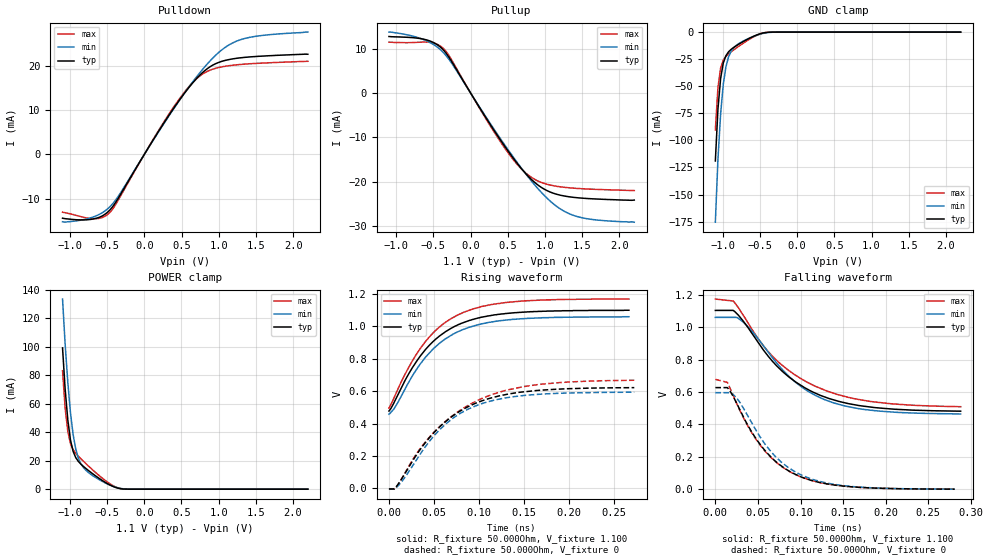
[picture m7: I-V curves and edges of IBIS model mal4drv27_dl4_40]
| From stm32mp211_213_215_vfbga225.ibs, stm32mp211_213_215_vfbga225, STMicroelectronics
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[Model] mal4drv27_dl4_40
Model_type   I/O
Polarity   Non-Inverting
Enable   Active-High
C_comp   1.656pF   1.654pF   1.662pF
C_comp_pullup   832.475fF   825.290fF   839.619fF
C_comp_pulldown 737.556fF   736.745fF   750.731fF
Vinh = 366.000mV
Vinl = 246.000mV
Vmeas = 306.000mV
Vref = 0.00V
Rref = 50Ohms
Cref = 0pF
[Model Spec]
Vinh   366.000mV   354.000mV   385.000mV
Vinl   246.000mV   234.000mV   265.000mV
Vmeas   306.000mV   294.000mV   325.000mV
Vref   0.00V   0.00V   0.00V
D_overshoot_ampl_h 0.3 NA   NA
D_overshoot_ampl_l 0.3 NA   NA
D_overshoot_area_l 100.000m NA   NA
D_overshoot_area_h 100.000m NA   NA
[Receiver Thresholds]
Vth = 306.000mV
Vth_min = 294.000mV
Vth_max = 325.000mV
Vinh_ac = 600.000mV
Vinh_dc = 600.000mV
Vinl_ac = -600.000mV
Vinl_dc = -600.000mV
Tslew_ac = 5.000ns
Threshold_sensitivity = 0.5
Reference_supply Pullup_ref
[Temperature Range]   25.000   125.000   -40.000
[Voltage Range]   1.100V   1.060V   1.170V
[GND Clamp Reference]   0.00V   0.00V   0.00V
[C Comp Corner]
| variable   typ   min   max
C_comp 1.662pF   1.656pF   1.654pF
C_comp_pullup 832.475fF   839.619fF   825.290fF
C_comp_pulldown 736.745fF   750.731fF   737.556fF
[Pulldown Reference]   0.00V   0.00V   0.00V
[POWER Clamp Reference]   1.100V   1.060V   1.170V
[Pullup Reference]   1.100V   1.060V   1.170V
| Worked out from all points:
|   slope of the pulldown table from 0 to 0.165 V, typ, clamps not added: 36.7 ohm
|   slope of the pullup table from 0 to 0.165 V, typ, clamps not added: 36.7 ohm
|   GND clamp passes 1 mA (typ) near -0.47 V on its own axis
|   POWER clamp passes 1 mA (typ) near -0.37 V on its own axis
|   rising waveform, R_fixture 50.000Ohm, V_fixture 1.100: 20-80 % time 53.2ps typ, 53ps min, 53.8ps max; typ from 0.478 V to 1.1 V
|   rising waveform, R_fixture 50.000Ohm, V_fixture 0: 20-80 % time 64.3ps typ, 59.5ps min, 73.7ps max; typ from -0.003 V to 0.622 V
|   falling waveform, R_fixture 50.000Ohm, V_fixture 1.100: 20-80 % time 71.3ps typ, 67.2ps min, 77.8ps max; typ from 1.1 V to 0.481 V
|   falling waveform, R_fixture 50.000Ohm, V_fixture 0: 20-80 % time 54.5ps typ, 54.4ps min, 54.9ps max; typ from 0.627 V to 0.001 V
[GND Clamp]
-1.099V   -119mA     -175.5mA   -90.46mA
-1.064V   -70.81mA   -117.3mA   -51.1mA
-1.028V   -42.76mA   -75.52mA   -33.21mA
-992.7mV  -28.64mA   -48.36mA   -25.94mA
-957.3mV  -21.83mA   -32.18mA   -22.47mA
-921.8mV  -18.22mA   -22.95mA   -20.16mA
-886.4mV  -15.9mA    -17.64mA   -18.21mA
-815.5mV  -12.5mA    -12.17mA   -14.62mA
-567.3mV  -3.324mA   -3.512mA   -3.774mA
-460.9mV  -879.1uA   -1.269mA   -863.6uA
-390mV    -181.5uA   -432.7uA   -123.2uA
2.198V    31.48nA    451.7nA    3.508nA
[Power Clamp]
-1.098V   99.1mA     133.3mA    83.09mA
-1.063V   70.06mA    101.6mA    56.85mA
-1.027V   48.48mA    74.82mA    40.4mA
-991.8mV  34.54mA    53.74mA    31.95mA
-956.4mV  26.58mA    38.45mA    27.74mA
-920.9mV  22.17mA    28.22mA    25.15mA
-885.5mV  19.46mA    21.74mA    23.1mA
-814.5mV  15.82mA    14.94mA    19.43mA
-743.6mV  12.83mA    11.41mA    15.93mA
-460mV    2.904mA    2.84mA     3.733mA
-282.7mV  117.7uA    274uA      108uA
2.199V    -10.68nA   -391.6nA   -2.283nA
[Pulldown]
-1.099V   -14.4mA    -15.2mA    -13.04mA
-673.6mV  -14.53mA   -14.04mA   -14.52mA
-567.3mV  -13.91mA   -13.19mA   -14.26mA
-460.9mV  -12.52mA   -11.78mA   -13.07mA
-319.1mV  -9.014mA   -8.658mA   -9.388mA
141.8mV   3.877mA    3.782mA    4.016mA
460.9mV   12mA       11.92mA    12.29mA
673.6mV   16.59mA    16.87mA    16.63mA
886.4mV   19.81mA    21.15mA    19.03mA
1.099V    21.26mA    24.3mA     19.92mA
1.312V    21.83mA    25.99mA    20.32mA
2.198V    22.6mA     27.6mA     21.01mA
[Pullup]
-1.098V   12.8mA     13.8mA     11.52mA
-637.3mV  12.21mA    12.14mA    11.54mA
-495.5mV  11.41mA    10.95mA    11.31mA
-389.1mV  10.15mA    9.549mA    10.43mA
-282.7mV  7.886mA    7.442mA    8.268mA
213.6mV   -5.793mA   -5.596mA   -6.04mA
532.7mV   -13.8mA    -13.53mA   -14.18mA
745.5mV   -18.3mA    -18.38mA   -18.15mA
958.2mV   -21.42mA   -22.61mA   -20.25mA
1.206V    -23.1mA    -26.21mA   -21.2mA
1.419V    -23.65mA   -27.86mA   -21.55mA
2.199V    -24.2mA    -29.2mA    -22.05mA
[Ramp]
R_load=50.000Ohm
dV/dt_r   373.440mV/59.500ps  357.809mV/57.500ps  400.680mV/65.500ps
dV/dt_f   373.440mV/64.500ps  357.809mV/62.500ps  400.680mV/68.000ps
[Rising waveform]
R_fixture=50.000Ohm
V_fixture=1.100
V_fixture_min=1.060
V_fixture_max=1.170
0s        477.8mV    458.7mV    496.4mV
9ps       568.3mV    521.4mV    602.3mV
20ps      688.3mV    635.9mV    727.2mV
30ps      779.2mV    729.7mV    823.4mV
39ps      846.3mV    798.5mV    895.4mV
60ps      956.3mV    912mV      1.014V
82ps      1.022V     980mV      1.085V
110ps     1.065V     1.024V     1.131V
148ps     1.088V     1.048V     1.157V
267ps     1.1V       1.06V      1.169V
[Rising waveform]
R_fixture=50.000Ohm
V_fixture=0
0s        -2.708mV   -4.143mV   -2.859mV
7ps       3.784mV    177.8uV    -2.859mV
15ps      66.75mV    47.29mV    68.05mV
33ps      227.4mV    198mV      233mV
57ps      383.6mV    365.8mV    385.3mV
76ps      466.6mV    452mV      470.7mV
96ps      525.2mV    509.1mV    536.2mV
128ps     577.9mV    557.5mV    603mV
166ps     605.4mV    581mV      641.9mV
273ps     622.3mV    594.2mV    668.1mV
[Falling waveform]
R_fixture=50.000Ohm
V_fixture=1.100
V_fixture_min=1.060
V_fixture_max=1.170
0s        1.103V     1.06V      1.173V
21ps      1.103V     1.06V      1.161V
32ps      1.042V     1.034V     1.08V
50ps      906.5mV    929.7mV    930.6mV
67ps      789.4mV    811.2mV    820.3mV
93ps      665.8mV    664.7mV    707mV
116ps     595.9mV    582.3mV    638.2mV
137ps     553.8mV    535.4mV    594.9mV
174ps     512.3mV    492.4mV    548.4mV
288ps     481.4mV    464.3mV    509.1mV
[Falling waveform]
R_fixture=50.000Ohm
V_fixture=0
0s        626.9mV    595.7mV    677.9mV
14ps      626.9mV    595.7mV    659.3mV
21ps      571.8mV    584.2mV    578.4mV
37ps      405.1mV    462.6mV    400.5mV
54ps      266.1mV    310.1mV    262.7mV
71ps      170.5mV    199.1mV    168.1mV
94ps      91.65mV    106.7mV    90.16mV
123ps     41.1mV     47.48mV    40.94mV
158ps     15.69mV    17.84mV    15.92mV
281ps     509uV      567.9uV    531.1uV
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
